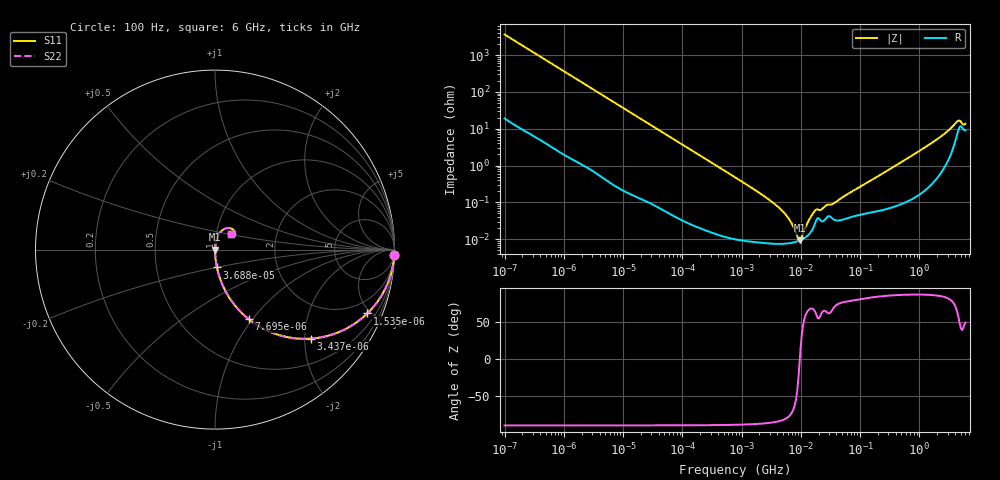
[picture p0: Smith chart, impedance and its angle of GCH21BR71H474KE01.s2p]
!Murata Part Number: GCH21BR71H474KE01
!These Parameters are Measured in Series Mode Connection
!Data Generated on Mar 13, 2026
!  o--ll--o
!Port1  Port2
!  o------o
!Operation Temp=25[degC], DC Bias Voltage=0[V]
!Freq. Start=100[Hz] Stop=6[GHz] 401[Steps]
# Hz S RI R 50
!Freq.(Hz) S11(Real) S11(Imag) S21(Real) S21(Imag) S12(Real) S12(Imag) S22(Real) S22(Imag)
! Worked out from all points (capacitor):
!   401 points, 100 Hz to 6 GHz, reference 50 ohm
!   read as one part in series: C = 439 nF near 109 Hz
!   lowest |Z| = 9.23 mohm at 9.506 MHz (marker M1)
!   series resonance near 9.63 MHz, so ESL is about 620 pH
!   S11 on the Smith chart (normalised r, x): 100 Hz: 1, -72; 1.535 kHz: 1.03, -4.76; 3.437 kHz: 1.01, -2.13; 7.695 kHz: 1.01, -0.96; 36.88 kHz: 1.00, -0.20; 6 GHz: 1.18, +0.20
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100  0.9991 -0.0276  0.000906 0.0276  0.000906 0.0276  0.9991 -0.0276
458  0.9838 -0.1237  0.0162 0.1237  0.0162 0.1237  0.9838 -0.1237
1535  0.8486 -0.3556  0.1514 0.3556  0.1514 0.3556  0.8486 -0.3556
2008  0.7672 -0.4197  0.2328 0.4197  0.2328 0.4197  0.7672 -0.4197
3437  0.5322 -0.496  0.4678 0.496  0.4678 0.496  0.5322 -0.496
7695  0.1873 -0.3874  0.8127 0.3874  0.8127 0.3874  0.1873 -0.3874
14402  0.0627 -0.2394  0.9373 0.2394  0.9373 0.2394  0.0627 -0.2394
36880  0.0107 -0.0992  0.9893 0.0992  0.9893 0.0992  0.0107 -0.0992
40335  0.00904 -0.0909  0.991 0.0909  0.991 0.0909  0.00904 -0.0909
774597  0.000122 -0.00481  0.9999 0.00481  0.9999 0.00481  0.000122 -0.00481
4440638  7.49e-05 -0.000675  0.9999 0.000675  0.9999 0.000675  7.49e-05 -0.000675
6353432  7.76e-05 -0.00034  0.9999 0.00034  0.9999 0.00034  7.76e-05 -0.00034
8692127  8.7e-05 -8.24e-05  0.9999 8.24e-05  0.9999 8.24e-05  8.7e-05 -8.24e-05
9506416  9.17e-05 -1.03e-05  0.9999 1.03e-05  0.9999 1.03e-05  9.17e-05 -1.03e-05
1.039699e7  9.79e-05 6.24e-05  0.9999 -6.24e-05  0.9999 -6.24e-05  9.79e-05 6.24e-05
1.555665e7  0.000178 0.000428  0.9998 -0.000428  0.9998 -0.000428  0.000178 0.000428
1.779312e7  0.000294 0.000546  0.9997 -0.000546  0.9997 -0.000546  0.000294 0.000546
3.64232e7  0.000339 0.000886  0.9997 -0.000886  0.9997 -0.000886  0.000339 0.000886
3.124326e8  0.000753 0.00782  0.9992 -0.00782  0.9992 -0.00782  0.000753 0.00782
1.873145e9  0.00628 0.0475  0.9937 -0.0475  0.9937 -0.0475  0.00628 0.0475
4.385646e9  0.084 0.1198  0.916 -0.1198  0.916 -0.1198  0.084 0.1198
6e9  0.0911 0.0853  0.9089 -0.0853  0.9089 -0.0853  0.0911 0.0853
